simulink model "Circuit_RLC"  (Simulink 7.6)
settings: Solver=ode15s  StartTime=0.0  StopTime=0.05  RelTol=1e-3
StopFcn:
  | close all
  | load tension_courant.mat
  | plotyy(ui(1,:),ui(3,:),ui(1,:),ui(4,:))
  | title('tension Vc de sortie et tension d''entrée')
  | xlabel('temps')
  | grid
  | 
  | 
  | figure
  | plotyy(ui(1,:),ui(2,:),ui(1,:),ui(4,:))
  | title('Courant dans le circuit et tension d''entrée')
  | xlabel('temps')
  | grid
libraries: fl_lib x13, nesl_utility x4

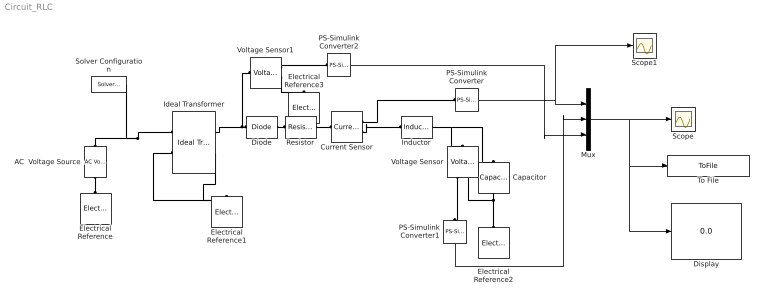
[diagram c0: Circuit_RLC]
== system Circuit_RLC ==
  AC  Voltage Source : fl_lib/Electrical/Electrical Sources/AC Voltage Source  DialogController=NetworkEngine.DynNeDlgSource  SystemSampleTime=-1  amp=220 V  shift=0 rad  omega=60 Hz  i_Log=off  v_Log=off  LocalVarNames=|i|v  LocalVarDescs=|i|v  LocalVarLogging=[0 0]
  Capacitor : fl_lib/Electrical/Electrical Elements/Capacitor  DialogController=NetworkEngine.DynNeDlgSource  SystemSampleTime=-1  c=1e-06 F  v0=0 V  r=1e-06 Ohm  g=0 1/Ohm  i_Log=off  v_Log=off  vc_Log=off  LocalVarNames=|i|v|vc  LocalVarDescs=|i|v|Internal variable for voltage across capacitor term  LocalVarLogging=[0 0 0]
  Current Sensor : fl_lib/Electrical/Electrical Sensors/Current Sensor  DialogController=NetworkEngine.DynNeDlgSource  SystemSampleTime=-1  i1_Log=off  v1_Log=off  LocalVarNames=|i1|v1  LocalVarDescs=|i1|v1  LocalVarLogging=[0 0]
  Diode : fl_lib/Electrical/Electrical Elements/Diode  DialogController=NetworkEngine.DynNeDlgSource  SystemSampleTime=-1  Vf=0.6 V  Ron=0.3 Ohm  Goff=1e-08 1/Ohm  i_Log=off  v_Log=off  LocalVarNames=|i|v  LocalVarDescs=|i|v  LocalVarLogging=[0 0]
  Display : Display
  Electrical Reference{,1..3} (4 alike) : fl_lib/Electrical/Electrical Elements/Electrical Reference  DialogController=NetworkEngine.DynNeDlgSource  SystemSampleTime=-1  i_Log=off  LocalVarNames=|i  LocalVarDescs=|i  LocalVarLogging=0
  Ideal Transformer : fl_lib/Electrical/Electrical Elements/Ideal Transformer  DialogController=NetworkEngine.DynNeDlgSource  SystemSampleTime=-1  n=220/12  i1_Log=off  v1_Log=off  i2_Log=off  v2_Log=off  LocalVarNames=|i1|v1|i2|v2  LocalVarDescs=|i1|v1|i2|v2  LocalVarLogging=[0 0 0 0]
  Inductor : fl_lib/Electrical/Electrical Elements/Inductor  DialogController=NetworkEngine.DynNeDlgSource  SystemSampleTime=-1  l=1e-3 H  i0=0 A  r=0 Ohm  g=1e-09 1/Ohm  i_Log=off  v_Log=off  i_L_Log=off  LocalVarNames=|i|v|i_L  LocalVarDescs=|i|v|Internal variable for current through inductor term  LocalVarLogging=[0 0 0]
  Mux : Mux  Inputs=3
  PS-Simulink Converter : nesl_utility/PS-Simulink Converter  DialogController=NetworkEngine.DynNeUtilDlgSource  SystemSampleTime=-1  PhysicalDomain=network_engine_domain  LeftPortType=input  RightPortType=output  SubClassName=ps_output  Unit=A  AffineConversion=off
  PS-Simulink Converter1 : nesl_utility/PS-Simulink Converter  DialogController=NetworkEngine.DynNeUtilDlgSource  SystemSampleTime=-1  PhysicalDomain=network_engine_domain  LeftPortType=input  RightPortType=output  SubClassName=ps_output  Unit=V  AffineConversion=off
  PS-Simulink Converter2 : nesl_utility/PS-Simulink Converter  DialogController=NetworkEngine.DynNeUtilDlgSource  SystemSampleTime=-1  PhysicalDomain=network_engine_domain  LeftPortType=input  RightPortType=output  SubClassName=ps_output  Unit=V  AffineConversion=off
  Resistor : fl_lib/Electrical/Electrical Elements/Resistor  DialogController=NetworkEngine.DynNeDlgSource  SystemSampleTime=-1  R=1 kOhm  i_Log=off  v_Log=off  LocalVarNames=|i|v  LocalVarDescs=|i|v  LocalVarLogging=[0 0]
  Scope : Scope
  Scope1 : Scope
  Solver Configuration : nesl_utility/Solver Configuration  DialogController=NetworkEngine.DynNeUtilDlgSource  SystemSampleTime=-1  PhysicalDomain=network_engine_domain  LeftPortType=input  RightPortType=generic  SubClassName=solver  Accelerate=off  Profile=off  ResidualTolerance=1e-9  MaxNonlinIter=12  MaxModeIter=2  DoFixedCost=off  UseLocalSampling=off  DoDC=off  LinearAlgebra=Sparse  LocalSolverSampleTime=.001  LocalSolverChoice=NE_BACKWARD_EULER_ADVANCER  UseLocalSolver=off
  To File : ToFile  Filename=tension_courant  MatrixName=ui
  Voltage Sensor : fl_lib/Electrical/Electrical Sensors/Voltage Sensor  DialogController=NetworkEngine.DynNeDlgSource  SystemSampleTime=-1  i1_Log=off  v1_Log=off  LocalVarNames=|i1|v1  LocalVarDescs=|i1|v1  LocalVarLogging=[0 0]
  Voltage Sensor1 : fl_lib/Electrical/Electrical Sensors/Voltage Sensor  DialogController=NetworkEngine.DynNeDlgSource  SystemSampleTime=-1  i1_Log=off  v1_Log=off  LocalVarNames=|i1|v1  LocalVarDescs=|i1|v1  LocalVarLogging=[0 0]
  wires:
  PS-Simulink Converter/1 -> Mux/1, Scope1/1
  PS-Simulink Converter1/1 -> Mux/2
  Mux/1 -> Scope/1, To File/1, Display/1
  PS-Simulink Converter2/1 -> Mux/3
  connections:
  AC  Voltage Source/RConn1 -- Electrical Reference/LConn1
  AC  Voltage Source/LConn1 -- Ideal Transformer/LConn1 -- Solver Configuration/RConn1
  Electrical Reference1/LConn1 -- Ideal Transformer/LConn2 -- Ideal Transformer/RConn2
  Inductor/LConn1 -- Capacitor/LConn1 -- Voltage Sensor/LConn1
  Capacitor/RConn1 -- Electrical Reference2/LConn1 -- Voltage Sensor/RConn2
  Current Sensor/LConn1 -- Resistor/RConn1
  Current Sensor/RConn2 -- Inductor/RConn1
  Current Sensor/RConn1 -- PS-Simulink Converter/LConn1
  Voltage Sensor/RConn1 -- PS-Simulink Converter1/LConn1
  Voltage Sensor1/RConn2 -- Electrical Reference3/LConn1
  Diode/LConn1 -- Voltage Sensor1/LConn1 -- Ideal Transformer/RConn1
  Voltage Sensor1/RConn1 -- PS-Simulink Converter2/LConn1
  Diode/RConn1 -- Resistor/LConn1
